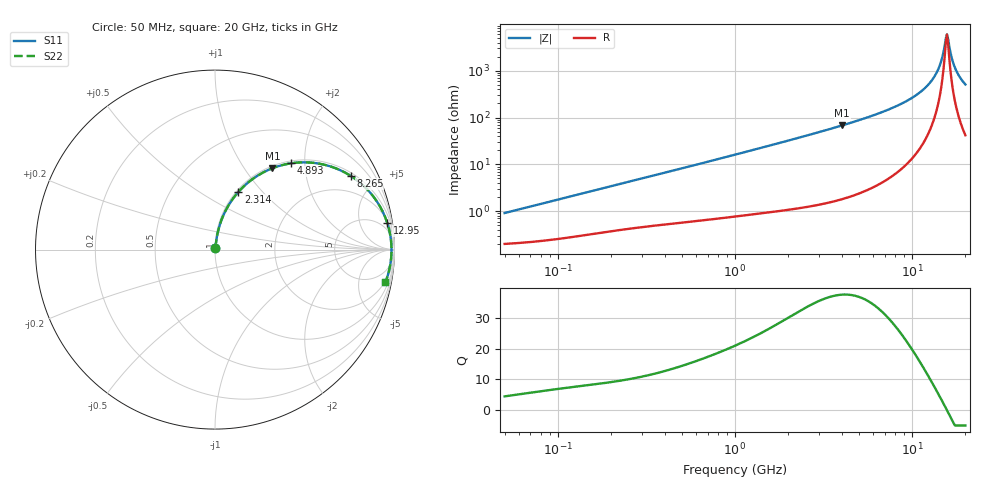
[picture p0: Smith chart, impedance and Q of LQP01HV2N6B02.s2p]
!Murata Part Number: LQP01HV2N6B02
!These Parameters are Measured in Series Mode Connection
!  o--[Z]--o
!Port1  Port2
!  o-------o
!Freq. Start=50[MHz] Stop=20[GHz], 401[Steps]
# Hz S RI R 50
!Freq.(Hz) S11(Real) S11(Imag) S21(Real) S21(Imag) S12(Real) S12(Imag) S22(Real) S22(Imag)
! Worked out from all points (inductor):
!   401 points, 50 MHz to 20 GHz, reference 50 ohm
!   read as one part in series: L = 2.83 nH near 51.52 MHz
!   highest Q = 37.6 at 4.027 GHz (marker M1), where L = 2.68 nH
!   self-resonance near 15.5 GHz
!   S11 on the Smith chart (normalised r, x): 50 MHz: 1.00, +0.02; 2.314 GHz: 1.02, +0.75; 4.893 GHz: 1.05, +1.71; 8.265 GHz: 1.14, +3.59; 12.95 GHz: 2, +13; 20 GHz: 2, -10
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5e7  0.00207 0.00888  0.9979 -0.00888  0.9979 -0.00888  0.00207 0.00888
1.364002e8  0.00355 0.0235  0.9964 -0.0235  0.9964 -0.0235  0.00355 0.0235
3.721004e8  0.0087 0.0605  0.9913 -0.0605  0.9913 -0.0605  0.0087 0.0605
1e9  0.0323 0.1545  0.9677 -0.1545  0.9677 -0.1545  0.0323 0.1545
2.313601e9  0.1304 0.3215  0.8696 -0.3215  0.8696 -0.3215  0.1304 0.3215
2.728004e9  0.172 0.3631  0.828 -0.3631  0.828 -0.3631  0.172 0.3631
4.026975e9  0.3202 0.4534  0.6798 -0.4534  0.6798 -0.4534  0.3202 0.4534
4.89267e9  0.4233 0.4808  0.5767 -0.4808  0.5767 -0.4808  0.4233 0.4808
7.442007e9  0.6888 0.4464  0.3112 -0.4464  0.3112 -0.4464  0.6888 0.4464
8.264682e9  0.7551 0.4116  0.2449 -0.4116  0.2449 -0.4116  0.7551 0.4116
1.082228e10  0.8989 0.2729  0.1011 -0.2729  0.1011 -0.2729  0.8989 0.2729
1.295331e10  0.9596 0.1489  0.0404 -0.1489  0.0404 -0.1489  0.9596 0.1489
1.417136e10  0.9764 0.0811  0.0236 -0.0811  0.0236 -0.0811  0.9764 0.0811
1.460232e10  0.9798 0.0579  0.0202 -0.0579  0.0202 -0.0579  0.9798 0.0579
1.527346e10  0.9828 0.023  0.0172 -0.023  0.0172 -0.023  0.9828 0.023
1.550395e10  0.9833 0.0113  0.0167 -0.0113  0.0167 -0.0113  0.9833 0.0113
1.573793e10  0.9835 -0.000441  0.0165 0.000441  0.0165 0.000441  0.9835 -0.000441
1.597544e10  0.9834 -0.0122  0.0166 0.0122  0.0166 0.0122  0.9834 -0.0122
1.696185e10  0.9802 -0.0589  0.0198 0.0589  0.0198 0.0589  0.9802 -0.0589
1.774144e10  0.9748 -0.0936  0.0252 0.0936  0.0252 0.0936  0.9748 -0.0936
1.88369e10  0.9639 -0.139  0.0361 0.139  0.0361 0.139  0.9639 -0.139
2e10  0.9488 -0.183  0.0512 0.183  0.0512 0.183  0.9488 -0.183
